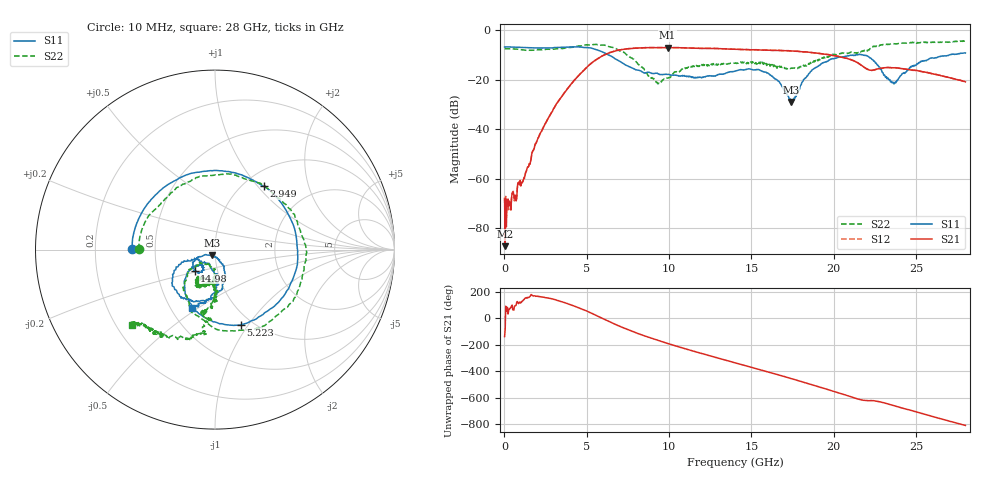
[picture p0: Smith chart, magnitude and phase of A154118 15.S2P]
!  2-Port S-parameters saved by WinCal
! VAR MeasName=S-Parameters (CALIBRATED_DATA) read from VNA (N5230A)
! VAR MeasDate=2015-9-10 14:35:28
! VAR NAME=A154118 15
! VAR FILENAME=A154118 15.S2P
! VAR DATE=2015-9-10 14:35:28
! VAR PHYS_PORTS=1,2
# Hz S DB R 50
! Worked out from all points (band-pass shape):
!   801 points, 10 MHz to 28 GHz, reference 50 ohm
!   highest |S21| = -6.94 dB at 9.911 GHz (marker M1); lowest = -87.1 dB at 44.99 MHz (marker M2)
!   |S21| within 3 dB of the highest: 6.06 GHz to 19.75 GHz (13.69 GHz wide, 106 % of centre)
!   lowest |S11| = -28.9 dB at 17.4 GHz (marker M3), VSWR 1.07, Z = 48.2 - j3.06 ohm
!   |S11| at or under -10 dB: 6.344 GHz to 21.14 GHz (14.8 GHz wide, 108 % of centre); 21.15 GHz to 21.33 GHz (187.9 MHz wide, 0.885 % of centre); 21.79 GHz to 27 GHz (5.211 GHz wide, 21.4 % of centre)
!   |S22| runs from -21.6 to -4.1 dB; largest |S21 - S12| = 0.0069
!   S11 on the Smith chart (normalised r, x): 10 MHz: 0.37, +0.00; 2.949 GHz: 1.22, +1.08; 5.223 GHz: 0.88, -0.92; 14.98 GHz: 0.78, -0.19; 28 GHz: 0.64, -0.47
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1e7  -6.74 179.6  -68.15 -137.1  -67.46 100.2  -7.49 179.8
4.49875e7  -6.72 178.3  -87.15 -84.4  -76.47 112.8  -7.46 178.7
1.1296e9  -6.95 134.7  -60.70 135.8  -60.85 137.2  -7.93 146.1
2.004288e9  -7.12 98.1  -44.02 168.2  -43.95 168.5  -7.84 122.3
2.94895e9  -7.03 52.5  -32.14 147.3  -32.12 147.6  -7.60 89.6
3.893612e9  -6.77 1.1  -22.98 108.9  -22.93 109.0  -6.92 51.7
4.698325e9  -6.79 -43.6  -16.97 70.9  -16.91 70.8  -6.24 12.5
5.223138e9  -7.06 -71.1  -13.61 42.8  -13.55 42.7  -5.90 -14.4
6.237775e9  -9.65 -115.1  -9.40 -16.2  -9.38 -16.4  -6.33 -67.4
7.532312e9  -14.52 -140.6  -7.40 -86.6  -7.37 -86.7  -10.50 -123.5
9.351662e9  -17.52 -138.9  -7.01 -167.0  -6.95 -167.3  -21.54 -115.0
9.911462e9  -17.79 -137.1  -6.94 171.0  -6.92 170.7  -19.27 -89.4
1.194074e10  -18.95 -127.9  -7.28 96.6  -7.26 96.1  -14.18 -103.8
1.4005e10  -16.52 -122.8  -7.65 24.4  -7.61 24.0  -13.26 -111.6
1.498465e10  -15.77 -134.3  -7.84 -8.5  -7.83 -9.2  -12.81 -113.3
1.613924e10  -18.07 -151.9  -8.03 -48.8  -8.02 -49.4  -14.47 -121.2
1.739879e10  -28.89 -118.3  -8.31 -94.0  -8.30 -94.7  -15.33 -109.5
1.869332e10  -15.96 -68.5  -8.99 -141.8  -8.99 -142.1  -12.47 -88.3
2.163228e10  -9.75 -127.0  -13.89 105.4  -13.91 104.3  -8.76 -99.5
2.334666e10  -19.97 -139.5  -14.99 71.8  -15.01 71.1  -5.66 -110.1
2.537594e10  -12.28 -88.7  -16.71 0.5  -16.71 0.3  -4.80 -126.9
2.8e10  -9.15 -111.6  -20.81 -88.9  -20.77 -89.0  -4.08 -137.7
